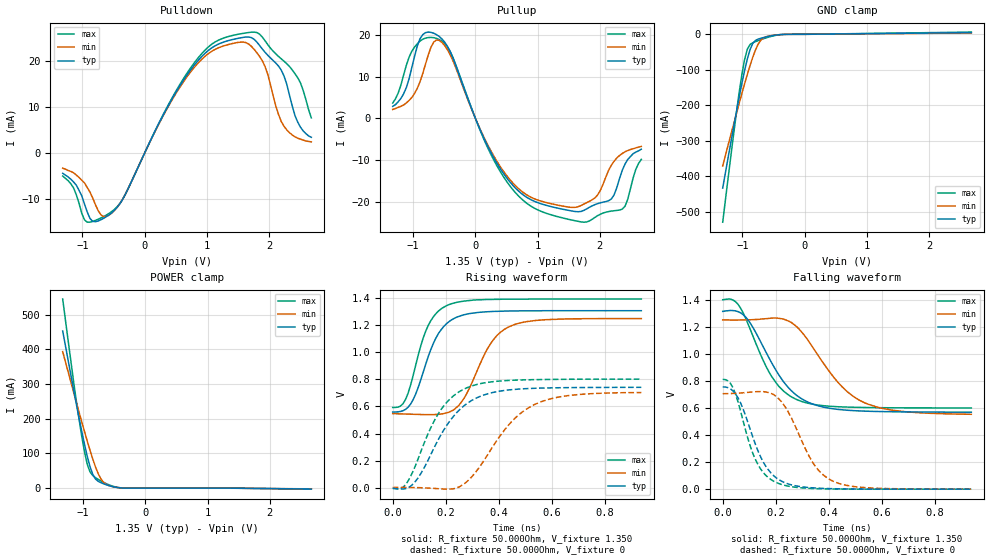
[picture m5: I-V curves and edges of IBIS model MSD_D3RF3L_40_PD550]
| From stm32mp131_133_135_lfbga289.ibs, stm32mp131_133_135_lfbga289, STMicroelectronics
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[Model] MSD_D3RF3L_40_PD550
Model_type   I/O
C_comp 2.422pF   2.338pF   2.546pF
Vinh = 810.000mV
Vinl = 540.000mV
Vmeas = 675.000mV
Vref = 675.000mV
[Model Spec]
Vinh   810.000mV   777.000mV   860.000mV
Vinl   540.000mV   507.000mV   590.000mV
Vmeas   675.000mV   642.000mV   725.000mV
Vref   675.000mV   642.000mV   725.000mV
[Receiver Thresholds]
Vth   =  0.675V
Vth_min  =  0.6615V
Vth_max  =  0.6885V
Vinh_ac  =  0.160V
Vinh_dc  =  0.090V
Vinl_ac  = -0.160V
Vinl_dc  = -0.090V
Tslew_ac =  5.000ns |Not specified, so set to high value
Threshold_sensitivity = 0.50
Reference_supply Pullup_ref
[Temperature Range]   25.000   125.000   -40.000
[Voltage Range]   1.350V   1.283V   1.450V
[GND Clamp Reference]   0.00V   0.00V   0.00V
[Pulldown Reference]   0.00V   0.00V   0.00V
[POWER Clamp Reference]   1.350V   1.283V   1.450V
[Pullup Reference]   1.350V   1.283V   1.450V
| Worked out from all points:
|   slope of the pulldown table from 0 to 0.203 V, typ, clamps not added: 35.6 ohm
|   slope of the pullup table from 0 to 0.203 V, typ, clamps not added: 29.7 ohm
|   GND clamp passes 1 mA (typ) near -0.40 V on its own axis
|   POWER clamp passes 1 mA (typ) near -0.41 V on its own axis
|   rising waveform, R_fixture 50.000Ohm, V_fixture 1.350: 20-80 % time 89.4ps typ, 110ps min, 77ps max; typ from 0.559 V to 1.31 V
|   rising waveform, R_fixture 50.000Ohm, V_fixture 0: 20-80 % time 143ps typ, 168ps min, 124ps max; typ from -0.005 V to 0.742 V
|   falling waveform, R_fixture 50.000Ohm, V_fixture 1.350: 20-80 % time 142ps typ, 170ps min, 120ps max; typ from 1.31 V to 0.568 V
|   falling waveform, R_fixture 50.000Ohm, V_fixture 0: 20-80 % time 94.9ps typ, 112ps min, 81.9ps max; typ from 0.755 V to 0 V
[GND Clamp]
-1.318V   -433.7mA   -371mA     -529.9mA
-1.142V   -261.3mA   -253.3mA   -281.1mA
-1.055V   -178.8mA   -195.8mA   -166mA
-1.011V   -139.6mA   -167.6mA   -114.8mA
-966.7mV  -102.8mA   -140.2mA   -71.91mA
-922.7mV  -69.98mA   -113.5mA   -42.24mA
-878.8mV  -43.33mA   -88.28mA   -28.82mA
-834.9mV  -25.71mA   -64.84mA   -23.86mA
-790.9mV  -17.19mA   -44.16mA   -20.64mA
-703mV    -11.03mA   -16.2mA    -14.94mA
-527.3mV  -4.003mA   -3.392mA   -5.338mA
2.68V     4.841mA    3.764mA    6.269mA
[Power Clamp]
-1.33V    452.9mA    393.3mA    544.8mA
-1.111V   242.4mA    247.7mA    251.5mA
-1.023V   162.7mA    190.7mA    148.6mA
-978.8mV  125.6mA    162.7mA    104mA
-934.9mV  91.47mA    135.5mA    68.54mA
-890.9mV  62.09mA    109.1mA    46.9mA
-847mV    39.75mA    84.16mA    36.4mA
-803mV    26.39mA    61.34mA    30.3mA
-715.1mV  15.71mA    26.57mA    20.81mA
-671.2mV  12.48mA    16.48mA    16.64mA
-407.6mV  908uA      1.189mA    1.109mA
2.668V    -2.431mA   -2.026mA   -2.89mA
[Pulldown]
-1.318V   -4.4mA     -3.3mA     -5mA
-922.7mV  -12.81mA   -7.5mA     -14.99mA
-703mV    -14.46mA   -13.41mA   -14.07mA
-571.2mV  -13.39mA   -13.44mA   -13.08mA
-351.5mV  -9.985mA   -9.964mA   -9.957mA
747mV     18.13mA    17.69mA    18.59mA
1.582V    25.03mA    24.01mA    25.9mA
1.889V    22.57mA    20.05mA    25.16mA
2.197V    17.93mA    6.8mA      20.38mA
2.329V    12.5mA     4.4mA      18.73mA
2.461V    6.7mA      3.2mA      16.3mA
2.68V     3.4mA      2.4mA      7.6mA
[Pullup]
-1.33V    2.9mA      2.152mA    3.679mA
-1.111V   7.4mA      3.715mA    12.77mA
-978.8mV  14.9mA     5.977mA    17.14mA
-715.1mV  20.68mA    17.1mA     19.47mA
-451.5mV  17.37mA    16.56mA    17.24mA
251.5mV   -8.249mA   -7.869mA   -8.718mA
866.7mV   -19.34mA   -18.75mA   -20.85mA
1.702V    -22.36mA   -20.93mA   -24.89mA
1.965V    -20.5mA    -18.41mA   -23.39mA
2.185V    -19.39mA   -11.29mA   -22.29mA
2.361V    -12.5mA    -8.438mA   -21.82mA
2.668V    -7.4mA     -6.748mA   -9.848mA
[Ramp]
R_load=50.000Ohm
dV/dt_r   444.420mV/117.000ps  422.039mV/140.000ps  478.740mV/100.500ps
dV/dt_f   444.420mV/118.500ps  422.039mV/143.000ps  478.740mV/101.500ps
[Rising waveform]
R_fixture=50.000Ohm
V_fixture=1.350
V_fixture_min=1.283
V_fixture_max=1.450
0s        558.7mV    546.7mV    592.6mV
39ps      568.7mV    544.6mV    620.9mV
68ps      619.2mV    542.8mV    761.6mV
135ps     974.2mV    539.4mV    1.203V
173ps     1.141V     542.1mV    1.306V
211ps     1.225V     556.8mV    1.352V
269ps     1.278V     659.5mV    1.379V
374ps     1.302V     1.078V     1.391V
441ps     1.306V     1.191V     1.393V
938ps     1.308V     1.25V      1.394V
[Rising waveform]
R_fixture=50.000Ohm
V_fixture=0
0s        -5.263mV   819.7uV    -4.884mV
48ps      -7.822mV   894.5uV    20.35mV
87ps      49.07mV    96.57uV    168.2mV
173ps     358.6mV    -8.328mV   549.3mV
230ps     528.5mV    -8.295mV   679.9mV
278ps     619mV      40.94mV    736.5mV
432ps     720.7mV    451mV      791.7mV
527ps     733.8mV    606.9mV    797.9mV
662ps     739.1mV    680.3mV    800.9mV
938ps     741.5mV    703mV      802mV
[Falling waveform]
R_fixture=50.000Ohm
V_fixture=1.350
V_fixture_min=1.283
V_fixture_max=1.450
0s        1.313V     1.25V      1.399V
48ps      1.317V     1.249V     1.385V
87ps      1.27V      1.25V      1.26V
183ps     939.2mV    1.263V     837.4mV
230ps     791.9mV    1.256V     723.4mV
278ps     694.2mV    1.202V     662.7mV
432ps     589.7mV    795.7mV    609.1mV
518ps     577.7mV    654.3mV    603.9mV
642ps     571.7mV    582.7mV    601mV
938ps     568.5mV    553.1mV    600mV
[Falling waveform]
R_fixture=50.000Ohm
V_fixture=0
0s        755.3mV    705mV      811mV
29ps      741.2mV    706.3mV    781.4mV
58ps      673.7mV    709.1mV    643.1mV
106ps     428.8mV    716.8mV    305.8mV
135ps     273.4mV    720.5mV    174.9mV
202ps     83.5mV     684.9mV    49.29mV
240ps     43.34mV    595.5mV    25.37mV
345ps     9.094mV    181.1mV    4.429mV
413ps     3.627mV    62.21mV    1.455mV
938ps     17uV       168.6uV    7.288uV
